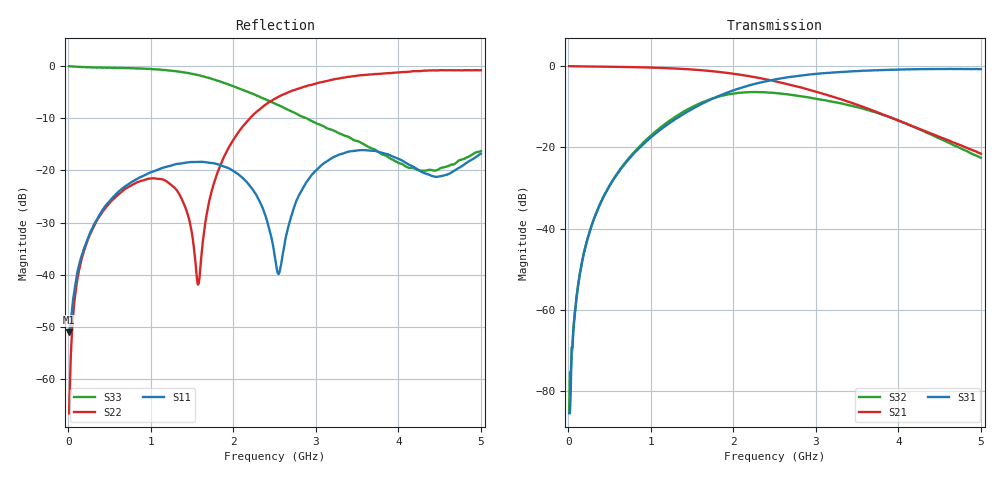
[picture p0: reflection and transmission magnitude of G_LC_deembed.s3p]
!AWR Design Environment (3650) Wed Dec 05 16:59:27 2007
!freq-unit  param-type  data-format  keyword  impedance-ohms
# GHz  S  DB  R  50
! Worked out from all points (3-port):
!   500 points, 10 MHz to 5 GHz, reference 50 ohm
!   strongest paths, dB at 10 MHz, 1.26 GHz, 2.51 GHz, 3.76 GHz, 5 GHz:
!     S31: -85.4, -13.6, -3.3, -1.0, -0.8
!     S21: 0.0, -0.6, -3.7, -11.4, -21.6
!     S32: -85.0, -13.0, -6.6, -11.6, -22.6
!   lowest |S11| = -51.0 dB at 10 MHz (marker M1), VSWR 1.01, Z = 50.3 + j0.0463 ohm
!   |S11| at or under -10 dB: start of sweep to end of sweep
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0.01  -51.01 9.4  -0.00 -0.4  -82.49 161.0
      -0.02 -0.4  -66.49 54.9  -80.55 124.0
      -85.38 -163.3  -84.95 -158.2  -0.06 179.2
0.07  -43.45 -42.4  -0.05 -2.6  -63.29 179.6
      -0.05 -2.7  -45.73 -53.0  -62.36 156.9
      -62.79 -177.0  -62.70 157.4  -0.14 175.7
0.18  -35.49 -70.4  -0.09 -6.6  -46.90 173.0
      -0.08 -6.5  -35.96 -67.8  -46.77 160.5
      -46.91 173.1  -46.93 160.5  -0.23 169.6
0.57  -24.67 -111.7  -0.19 -20.3  -27.20 158.8
      -0.19 -20.2  -25.15 -89.7  -27.10 142.3
      -27.20 158.9  -27.08 142.3  -0.37 148.7
1.29  -18.86 -160.0  -0.60 -47.4  -13.17 132.6
      -0.59 -47.3  -23.37 -125.7  -12.55 93.3
      -13.14 132.5  -12.57 93.1  -0.99 99.7
1.57  -18.37 -176.8  -0.95 -59.2  -9.77 121.0
      -0.95 -59.0  -41.87 144.0  -9.39 69.1
      -9.81 121.1  -9.40 69.0  -1.74 73.7
1.86  -19.10 166.7  -1.52 -71.9  -7.03 108.0
      -1.52 -71.9  -18.36 25.8  -7.34 41.9
      -7.02 108.0  -7.31 41.8  -3.12 43.2
2.51  -37.28 169.7  -3.72 -100.6  -3.26 78.3
      -3.72 -100.3  -6.26 -18.2  -6.62 -14.3
      -3.26 78.6  -6.62 -14.6  -7.29 -14.0
3.22  -17.43 -98.7  -7.63 -127.4  -1.55 52.0
      -7.61 -127.7  -2.57 -55.4  -8.83 -61.5
      -1.56 51.9  -8.83 -61.3  -12.42 -24.0
5  -16.80 -59.6  -21.39 -160.2  -0.60 9.4
   -21.57 -160.3  -0.85 -132.1  -22.65 -143.9
   -0.75 9.5  -22.56 -143.7  -16.30 -99.7
